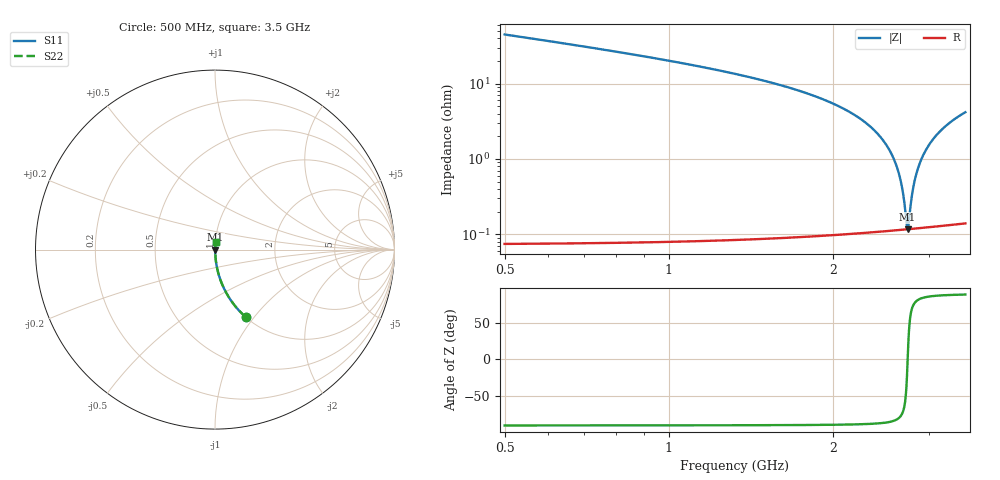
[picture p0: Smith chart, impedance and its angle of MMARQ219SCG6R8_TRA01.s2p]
! MMARQ219SCG6R8_TRA01  S-PARAMETER MODEL  ( General Type )
! Model Generated by TAIYO YUDEN Corporation (http://www.ty-top.com)
! Version 1.0
! TAIYO YUDEN Control No. 180601
! Copyright(c) 2018 TAIYO YUDEN CO.,LTD. All Rights Reserved.
! Product Description (link to TY-COMPAS)
! https://ds.yuden.co.jp/TYCOMPAS/or/detail?pn=MMARQ219SCG6R8CTRA01&u=M
! Products Name : Multilayer Ceramic Capacitors
! Characteristics :
!  Capacitance : 6.8 pF , Rated Voltage : 250V , TCC : CG / C0G
!  Case Size : 2.0 x 1.25 / 0.079 x 0.049 [mm/inch] , Thickness : 0.85 / 0.033 [mm/inch]
!  (Conditions: Temperature = 25 degC , DC Bias Current/Voltage = 0A / 0V)
! External Node Assignments :
!  1  o---| |---o  2
! GND o---------o GND
! Frequency Range : 500MHz  -  3500MHz  [ 401 STEP ]
# MHz S RI R 50
! Freq[MHz].  S11 Real  S11 Imag  S21 Real  S21 Imag  S12 Real  S12 Imag  S22 Real  S22 Imag
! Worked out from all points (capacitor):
!   401 points, 500 MHz to 3.5 GHz, reference 50 ohm
!   read as one part in series: C = 6.8 pF near 515 MHz
!   lowest |Z| = 117 mohm at 2.743 GHz (marker M1)
!   series resonance near 2.743 GHz, so ESL is about 490 pH
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500  0.1702 -0.375  0.8298 0.375  0.8298 0.375  0.1702 -0.375
710  0.0869 -0.2804  0.9131 0.2804  0.9131 0.2804  0.0869 -0.2804
1002.5  0.0399 -0.1939  0.9601 0.1939  0.9601 0.1939  0.0399 -0.1939
1505  0.0125 -0.1071  0.9875 0.1071  0.9875 0.1071  0.0125 -0.1071
2000  0.00395 -0.0544  0.9961 0.0544  0.9961 0.0544  0.00395 -0.0544
2300  0.00195 -0.0301  0.998 0.0301  0.998 0.0301  0.00195 -0.0301
2412.5  0.00155 -0.0219  0.9984 0.0219  0.9984 0.0219  0.00155 -0.0219
2502.5  0.00134 -0.0156  0.9987 0.0156  0.9987 0.0156  0.00134 -0.0156
2585  0.00122 -0.0101  0.9988 0.0101  0.9988 0.0101  0.00122 -0.0101
2645  0.00118 -0.00617  0.9988 0.00617  0.9988 0.00617  0.00118 -0.00617
2682.5  0.00116 -0.00378  0.9988 0.00378  0.9988 0.00378  0.00116 -0.00378
2705  0.00116 -0.00236  0.9988 0.00236  0.9988 0.00236  0.00116 -0.00236
2727.5  0.00116 -0.000948  0.9988 0.000948  0.9988 0.000948  0.00116 -0.000948
2742.5  0.00117 -1.63e-05  0.9988 1.63e-05  0.9988 1.63e-05  0.00117 -1.63e-05
2757.5  0.00117 0.00091  0.9988 -0.00091  0.9988 -0.00091  0.00117 0.00091
2787.5  0.00119 0.00275  0.9988 -0.00275  0.9988 -0.00275  0.00119 0.00275
2802.5  0.0012 0.00366  0.9988 -0.00366  0.9988 -0.00366  0.0012 0.00366
2847.5  0.00124 0.00637  0.9988 -0.00637  0.9988 -0.00637  0.00124 0.00637
2915  0.00132 0.0103  0.9987 -0.0103  0.9987 -0.0103  0.00132 0.0103
3005  0.00148 0.0155  0.9985 -0.0155  0.9985 -0.0155  0.00148 0.0155
3215  0.00204 0.0271  0.998 -0.0271  0.998 -0.0271  0.00204 0.0271
3500  0.00314 0.0417  0.9969 -0.0417  0.9969 -0.0417  0.00314 0.0417
